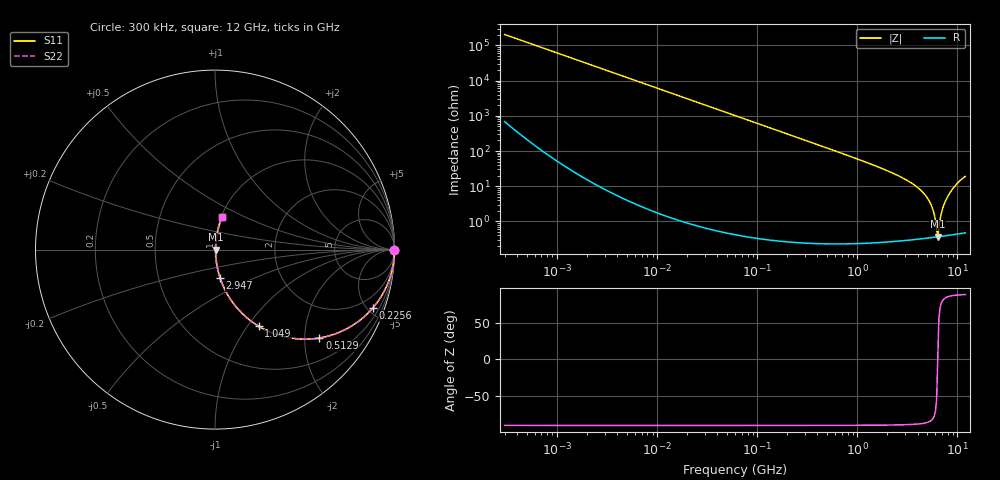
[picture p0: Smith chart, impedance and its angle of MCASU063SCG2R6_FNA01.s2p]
! MCASU063SCG2R6_FNA01  S-PARAMETER MODEL  ( General Type )
! Model Generated by TAIYO YUDEN Corporation (http://www.ty-top.com)
! Version 1.0
! TAIYO YUDEN Control No. 130801
! Copyright(c) 2013 TAIYO YUDEN CO.,LTD. All Rights Reserved.
! Product Description (link to TY-COMPAS)
! https://ds.yuden.co.jp/TYCOMPAS/or/detail?pn=MCASU063SCG2R6CFNA01&u=M
! Products Name : Multilayer Ceramic Capacitors
! Characteristics :
!  Capacitance : 2.6 pF , Rated Voltage : 50V , TCC : CG / C0G
!  Case Size : 0.6 x 0.3 / 0.024 x 0.012 [mm/inch] , Thickness : 0.3 / 0.012 [mm/inch]
!  (Conditions: Temperature = 25 degC , DC Bias Current/Voltage = 0A / 0V)
! External Node Assignments :
!  1  o---| |---o  2
! GND o---------o GND
! Frequency Range : 0.3MHz  -  12000MHz  [ 401 STEP ]
# MHz S RI R 50
! Freq[MHz].  S11 Real  S11 Imag  S21 Real  S21 Imag  S12 Real  S12 Imag  S22 Real  S22 Imag
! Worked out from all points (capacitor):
!   401 points, 300 kHz to 12 GHz, reference 50 ohm
!   read as one part in series: C = 2.61 pF near 316.3 kHz
!   lowest |Z| = 367 mohm at 6.354 GHz (marker M1)
!   series resonance near 6.349 GHz, so ESL is about 240 pH
!   S11 on the Smith chart (normalised r, x): 300 kHz: open; 225.6 MHz: 1.01, -5.40; 512.9 MHz: 1.00, -2.36; 1.049 GHz: 1.00, -1.13; 2.947 GHz: 1.01, -0.32; 12 GHz: 1.01, +0.38
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0.3  1 -0.000492  1.9e-06 0.000492  1.9e-06 0.000492  1 -0.000492
1.769972  1 -0.0029  1e-05 0.0029  1e-05 0.0029  1 -0.0029
10.44266  0.9997 -0.0171  0.000298 0.0171  0.000298 0.0171  0.9997 -0.0171
60  0.9904 -0.0975  0.00964 0.0975  0.00964 0.0975  0.9904 -0.0975
225.6362  0.8789 -0.3257  0.1211 0.3257  0.1211 0.3257  0.8789 -0.3257
353.9943  0.7463 -0.4345  0.2537 0.4345  0.2537 0.4345  0.7463 -0.4345
512.9422  0.582 -0.4922  0.418 0.4922  0.418 0.4922  0.582 -0.4922
1048.836  0.2431 -0.4268  0.7569 0.4268  0.7569 0.4268  0.2431 -0.4268
2088.533  0.0656 -0.2426  0.9344 0.2426  0.9344 0.2426  0.0656 -0.2426
2947.191  0.0283 -0.1573  0.9717 0.1573  0.9717 0.1573  0.0283 -0.1573
3944.255  0.012 -0.0936  0.988 0.0936  0.988 0.0936  0.012 -0.0936
4875.354  0.00594 -0.051  0.9941 0.051  0.9941 0.051  0.00594 -0.051
5565.855  0.00413 -0.0254  0.9959 0.0254  0.9959 0.0254  0.00413 -0.0254
6026.253  0.00369 -0.0102  0.9963 0.0102  0.9963 0.0102  0.00369 -0.0102
6188.031  0.00364 -0.00511  0.9964 0.00511  0.9964 0.00511  0.00364 -0.00511
6354.153  0.00365 0.000174  0.9963 -0.000174  0.9963 -0.000174  0.00365 0.000174
6524.734  0.00372 0.00539  0.9963 -0.00539  0.9963 -0.00539  0.00372 0.00539
6699.894  0.00384 0.0105  0.9962 -0.0105  0.9962 -0.0105  0.00384 0.0105
7254.098  0.00458 0.0272  0.9954 -0.0272  0.9954 -0.0272  0.00458 0.0272
8064.993  0.00679 0.0526  0.9932 -0.0526  0.9932 -0.0526  0.00679 0.0526
9708.23  0.0164 0.1088  0.9836 -0.1088  0.9836 -0.1088  0.0164 0.1088
12000  0.0392 0.182  0.9608 -0.182  0.9608 -0.182  0.0392 0.182
